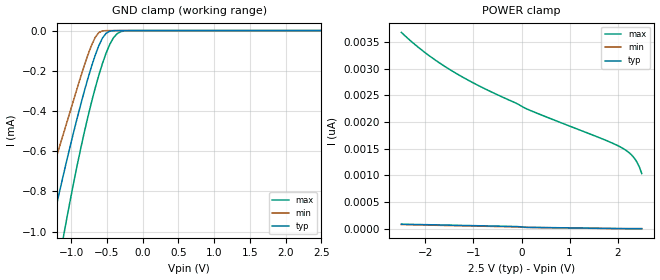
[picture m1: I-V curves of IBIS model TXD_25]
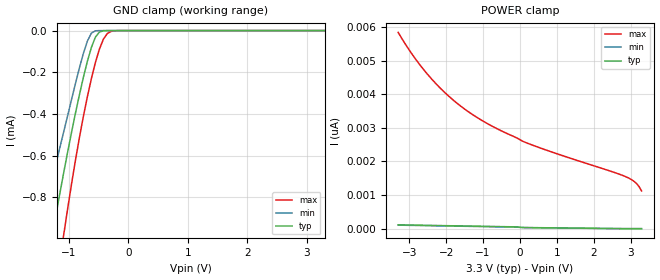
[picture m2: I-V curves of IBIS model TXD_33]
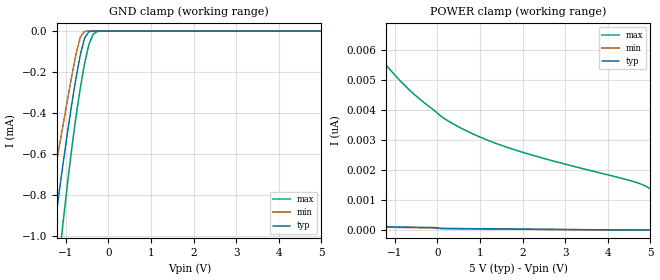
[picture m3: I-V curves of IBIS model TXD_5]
| IBIS file created by Layout Workbench Version 22.1.4.12161.401368   004
| Cadence Design Systems, Inc. 2011
[IBIS ver]   4.2
[File name]  iso64xx.ibs
[File Rev]   1.5
[Date]   05 15, 2025
[Source]   Model built from TISPICED simulations at:
   Texas Instruments Incorporated.
   Analog-eLab, HPA 12500 TI Blvd
   Dallas, TX -75243
   For Support e-mail: elab_ibis@list.ti.com
[Notes]   This product is designed as an aid for customers of Texas Instruments.
   No warranties, either expressed or implied, with respect to this third party software (if any)
   or with respect to its fitness for any particular purpose is claimed by Texas Instruments or
   the author. The software (if any) is provided solely on an "as is" basis. The entire risk as to
   its quality and performance is with the customer
[Disclaimer]  This product is designed as an aid for customers of Texas Instruments. No warranties, either expressed or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
[Copyright] (C)Copyright 2025 Texas Instruments Incorporated. All rights reserved.
|   Component ISO64XX
[Component] ISO6441DW
[Manufacturer] Texas Instruments Incorporated
[Package]   |16-pin SOIC DW package
|   typ   min   max
R_pkg   0.04817   0.03432   0.09530
L_pkg   2.4595nH   1.6904nH   4.7034nH
C_pkg   0.847pF   0.428pF   1.397pF
[Pin]  signal_name   model_name   R_pin   L_pin   C_pin
1   VCC1   POWER   0.03455  3.39778n  0.89677p
2   GND1   GND   0.03432  3.12613n  0.84706p
3   INA   TXD1   0.04265  1.85523n  0.57831p
4   INB   TXD1   0.03948  1.69049n  0.59300p
5   INC   TXD1   0.03943  1.70546n  0.55709p
6   OUTD   RXD1   0.04257  1.86953n  0.56379p
7   EN1   TXDM1   0.04783  1.99000n  0.60148p
8   GND1   GND   0.03740  4.70338n  1.39696p
9   GND2   GND   0.03763  4.61305n  1.39587p
10   EN2   TXDM1   0.04703  2.01514n  0.58483p
11   IND   TXD2   0.07132  2.45946n  0.43321p
12   OUTC   RXD2   0.06147  2.13194n  0.42769p
13   OUTB   RXD2   0.07288  2.39260n  0.48001p
14   OUTA   RXD2   0.09530  3.03704n  0.47622p
15   GND2   GND   0.04817  4.23145n  0.93567p
16   VCC2   POWER   0.04790  4.51154n  0.99405p
[Model Selector] TXD1
TXD_25   TXD Input model for 2.25V - 2.75V
TXD_33   TXD Input model for 3.0V - 3.6V
TXD_5   TXD Input model for 4.5V - 5.5V
[Model Selector] RXD1
RXD_25   RXD Output model for 2.25V - 2.75V
RXD_33   RXD Output model for 3.0V - 3.6V
RXD_5   RXD Output model for 4.5V - 5.5V
[Model Selector] TXDM1
TXDM_25   TXD Input model for 2.25V - 2.75V
TXDM_33   TXD Input model for 3.15V - 3.6V
TXDM_5   TXD Input model for 4.5V - 5.5V
[Model Selector] TXD2
TXD_25   TXD Input model for 2.25V - 2.75V
TXD_33   TXD Input model for 3.0V - 3.6V
TXD_5   TXD Input model for 4.5V - 5.5V
[Model Selector] RXD2
RXD_25   RXD Output model for 2.25V - 2.75V
RXD_33   RXD Output model for 3.0V - 3.6V
RXD_5   RXD Output model for 4.5V - 5.5V
| Models and submodels in the file (9): TXD_25 (Input), TXD_33 (Input), TXD_5 (Input), TXDM_25 (Input), TXDM_33 (Input), TXDM_5 (Input), RXD_25 (3-state), RXD_33 (3-state), RXD_5 (3-state)
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|   TXD_25 Model
[Model]   TXD_25
Model_type   Input
|Signals   TXD
Vinl =  0.750V
Vinh =  1.750V
|   typ   min   max
C_comp   1.3pF   1.1pF   1.5pF
|   typ   min   max
[Temperature Range]   27   -40   125
[Voltage range]   2.5V   2.25V   2.75V
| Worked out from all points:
|   GND clamp passes 1 mA (typ) near -1.29 V on its own axis
[GND_clamp]
|Voltage   I(typ)   I(min)   I(max)
-2.5V     -3.261mA   -2.697mA   -4.025mA
-1.48V    -1.333mA   -1.01mA    -1.787mA
-1.276V   -983uA     -716.4uA   -1.36mA
-1.123V   -739.3uA   -529.9uA   -1.053mA
-1.072V   -661.5uA   -470.4uA   -954.6uA
-919mV    -439.5uA   -290uA     -675.2uA
-766mV    -238.2uA   -120.7uA   -428.7uA
-613mV    -74.62uA   -9.78uA    -221.8uA
-511mV    -13.26uA   -161.8nA   -111.7uA
-409mV    -630.3nA   -1.04nA    -36.14uA
-256mV    -2.009nA   -6.036pA   -1.659uA
2.5V      0A         0A         0A
[POWER_clamp]
|Voltage   I(typ)   I(min)   I(max)
-2.5V     84.61pA    76.91pA    3.684nA
-2.192V   78.79pA    71.19pA    3.438nA
-1.835V   72.09pA    64.59pA    3.191nA
-1.427V   64.46pA    57.09pA    2.951nA
-1.019V   56.88pA    49.63pA    2.744nA
154mV     24.79pA    22.52pA    2.229nA
1.684V    6.302pA    4.156pA    1.684nA
2.092V    1.394pA    0A         1.515nA
2.245V    0A         0A         1.42nA
2.347V    0A         0A         1.323nA
2.449V    0A         0A         1.162nA
2.5V      0A         0A         1.034nA
|   TXD_33 Model
[Model]   TXD_33
Model_type   Input
|Signals   TXD
Vinl =  0.990V
Vinh =  2.310V
|   typ   min   max
C_comp   1.3pF   1.1pF   1.5pF
|   typ   min   max
[Temperature Range]   27   -40   125
[Voltage range]   3.3V   3.0V   3.6V
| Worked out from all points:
|   GND clamp passes 1 mA (typ) near -1.29 V on its own axis
[GND_clamp]
|Voltage   I(typ)   I(min)   I(max)
-3.3V     -4.822mA   -4.059mA   -5.82mA
-1.491V   -1.352mA   -1.027mA   -1.81mA
-1.424V   -1.234mA   -925uA     -1.668mA
-1.29V    -1.006mA   -734.8uA   -1.389mA
-1.223V   -896.7uA   -649.1uA   -1.252mA
-1.089V   -687.3uA   -490.2uA   -987.2uA
-754mV    -223.6uA   -108.8uA   -410.9uA
-620mV    -80.65uA   -12.05uA   -230.3uA
-553mV    -31.67uA   -1.049uA   -153.7uA
-419mV    -886.2nA   -1.734nA   -41.6uA
-218mV    -449.6pA   -6.494pA   -628.3nA
3.3V      0A         0A         0A
[POWER_clamp]
|Voltage   I(typ)   I(min)   I(max)
-3.3V     113.7pA    104.6pA    5.836nA
-3.065V   109.2pA    100.1pA    5.419nA
-2.797V   104pA      95.04pA    4.996nA
-2.328V   94.97pA    86.22pA    4.372nA
-1.792V   84.76pA    76.21pA    3.81nA
-1.256V   74.65pA    66.26pA    3.373nA
-720mV    64.61pA    56.39pA    3.029nA
151mV     33.16pA    30.36pA    2.565nA
2.898V    0A         0A         1.532nA
3.166V    0A         0A         1.339nA
3.233V    0A         0A         1.249nA
3.3V      0A         0A         1.12nA
|   TXD_5 Model
[Model]   TXD_5
Model_type   Input
|Signals   TXD
Vinl =  1.500V
Vinh =  3.500V
|   typ   min   max
C_comp   1.3pF   1.1pF   1.5pF
|   typ   min   max
[Temperature Range]   27   -40   125
[Voltage range]   5.0V   4.5V   5.5V
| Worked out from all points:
|   GND clamp passes 1 mA (typ) near -1.29 V on its own axis
[GND_clamp]
|Voltage   I(typ)   I(min)   I(max)
-5V       -8.158mA   -6.968mA   -9.644mA
-1.465V   -1.306mA   -987uA     -1.755mA
-1.263V   -961.6uA   -699.5uA   -1.333mA
-1.162V   -799.9uA   -575.6uA   -1.13mA
-1.061V   -645uA     -457.5uA   -933.6uA
-758mV    -228.5uA   -112.7uA   -416.8uA
-657mV    -115.6uA   -29.62uA   -276.8uA
-556mV    -33.38uA   -1.189uA   -156.8uA
-455mV    -2.832uA   -10.7nA    -64.96uA
-354mV    -87.76nA   -69.95pA   -14.52uA
-253mV    -1.79nA    -9.666pA   -1.545uA
5V        0A         0A         0A
[POWER_clamp]
|Voltage   I(typ)   I(min)   I(max)
-5V       179.5pA    164pA      20.45nA
-1.868V   115.6pA    102.9pA    6.803nA
-1.767V   113.6pA    101pA      6.576nA
-1.262V   103.8pA    91.4pA     5.583nA
-757mV    94.06pA    81.91pA    4.792nA
51mV      56.19pA    49.29pA    3.815nA
455mV     46.94pA    42.18pA    3.461nA
1.061V    39.62pA    34.91pA    3.053nA
1.768V    31.11pA    26.43pA    2.686nA
2.677V    20.17pA    15.53pA    2.309nA
4.596V    0A         0A         1.612nA
5V        0A         0A         1.364nA
